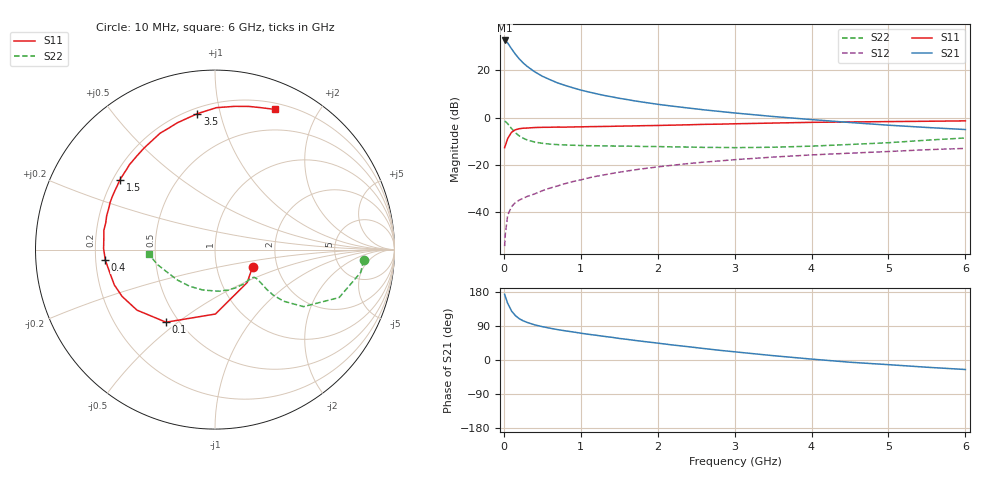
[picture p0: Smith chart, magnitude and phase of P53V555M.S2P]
! SIEMENS Small Signal Semiconductors
! BFP183
! Si NPN RF Bipolar Junction Transistor in SOT143
! VCE = 3.5 V  IC = 55 mA
! Common Emitter S-Parameters:  March  1996
# GHz  S  MA  R  50
!  f  S11  S21  S12  S22
! GHz  MAG  ANG  MAG  ANG  MAG  ANG  MAG  ANG
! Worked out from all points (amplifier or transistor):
!   36 points, 10 MHz to 6 GHz, reference 50 ohm
!   highest |S21| = 32.6 dB at 10 MHz (marker M1)
!   |S21| within 3 dB of that: start of sweep to 89.38 MHz
!   unconditionally stable (mu >= 1): start of sweep to 20.11 MHz; 287.3 MHz to end of sweep
!   at 250 MHz: K = 0.92, MSG = 28.7 dB, |S12| = -34.2 dB
!   at 1.4 GHz: K = 1.44, MAG = 12.3 dB, |S12| = -23.7 dB
!   at 6 GHz: K = 1.10, MAG = 2.1 dB, |S12| = -13.1 dB
!   S11 on the Smith chart (normalised r, x): 10 MHz: 1.49, -0.30; 100 MHz: 0.43, -0.45; 400 MHz: 0.24, -0.04; 1.5 GHz: 0.23, +0.31; 3.5 GHz: 0.23, +0.85; 6 GHz: 0.26, +1.48
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0.01  0.2305 -24.7  42.68 173.4  0.0019 74.6  0.8306 -4.1
0.02  0.2565 -45.6  42.14 167.2  0.0035 76.4  0.8216 -8.9
0.05  0.3589 -89.6  37.78 149.5  0.0086 67.7  0.7416 -21.1
0.1  0.488 -124.0  28.45 129.4  0.013 54.0  0.5865 -32.8
0.15  0.5502 -142.2  21.88 117.1  0.0159 49.8  0.4772 -37.0
0.2  0.5795 -153.2  17.43 109.1  0.0179 49.9  0.4088 -38.0
0.25  0.5945 -160.7  14.36 103.5  0.0195 49.9  0.3661 -37.6
0.3  0.5984 -166.3  12.18 99.4  0.0213 53.0  0.3369 -36.7
0.4  0.6141 -174.6  9.304 92.8  0.0242 54.4  0.3031 -35.5
0.5  0.6206 179.5  7.479 88.0  0.0283 56.7  0.285 -34.9
0.6  0.6224 174.4  6.314 83.9  0.0322 58.4  0.2739 -34.9
0.7  0.6283 170.1  5.389 80.2  0.0358 60.6  0.267 -35.3
0.9  0.6322 162.7  4.244 74.0  0.0443 60.9  0.2592 -37.6
1.1  0.6407 155.7  3.482 67.8  0.0528 61.3  0.2535 -40.6
1.5  0.6576 143.6  2.555 56.9  0.0697 59.4  0.249 -48.3
1.8  0.6717 135.2  2.126 49.3  0.0822 57.7  0.2444 -55.5
2.2  0.6903 124.9  1.733 39.5  0.0981 54.0  0.2391 -65.8
2.8  0.7241 110.9  1.348 25.7  0.1207 48.0  0.233 -83.9
3.5  0.7637 97.4  1.051 11.5  0.1455 41.3  0.2353 -107.3
4.5  0.8058 82.1  0.785 -5.9  0.1762 31.3  0.2691 -140.8
5.5  0.8335 71.3  0.616 -19.1  0.2086 22.6  0.3321 -165.6
6  0.8496 66.8  0.557 -25.1  0.2222 17.5  0.3697 -176.1
